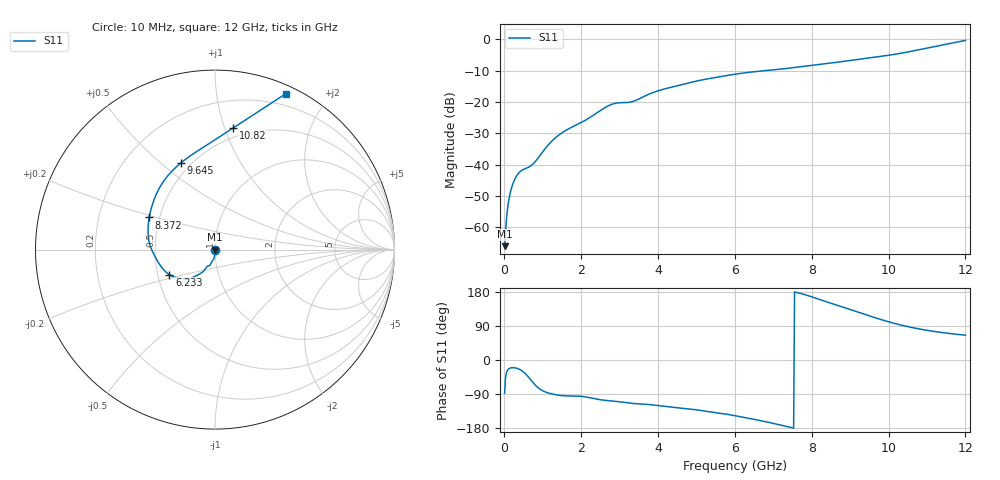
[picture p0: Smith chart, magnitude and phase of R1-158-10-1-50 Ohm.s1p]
!version-1
!date-10.2020
!Series
#GHZ	S	RI	R	50.0
!FREQ.GHZ	S11RE	S11IM
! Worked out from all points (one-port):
!   500 points, 10 MHz to 12 GHz, reference 50 ohm
!   lowest |S11| = -66.0 dB at 10 MHz (marker M1), VSWR 1.00, Z = 50 - j0.05 ohm
!   |S11| at or under -10 dB: start of sweep to 6.819 GHz
!   S11 on the Smith chart (normalised r, x): 10 MHz: 1.00, -0.00; 6.233 GHz: 0.58, -0.17; 8.372 GHz: 0.44, +0.19; 9.645 GHz: 0.44, +0.58; 10.82 GHz: 0.42, +1.07; 12 GHz: 0.08, +1.55
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0.01  2e-05 -0.0005
0.0340281  0.000576 -0.000622
0.0820842  0.00167 -0.00087
0.106112  0.00221 -0.000998
0.13014  0.00274 -0.00113
0.202224  0.00421 -0.00156
0.298337  0.00583 -0.00225
0.442505  0.0071 -0.00365
0.75487  0.00512 -0.00896
1.18737  0.00069 -0.022
1.52377  -0.00235 -0.0327
2.10044  -0.00628 -0.0501
2.70114  -0.0254 -0.0824
3.01351  -0.0338 -0.0911
3.3499  -0.0425 -0.0926
3.92657  -0.071 -0.1264
4.52727  -0.1078 -0.1473
5.07992  -0.1492 -0.1623
6.01701  -0.2331 -0.1502
6.23327  -0.2542 -0.1389
6.858  -0.3057 -0.0871
7.50675  -0.351 -0.00485
8.37176  -0.3667 0.1792
9.02052  -0.3119 0.339
9.64525  -0.1922 0.4813
10.5103  0.0237 0.6272
10.8226  0.1016 0.6781
12  0.396 0.8697
